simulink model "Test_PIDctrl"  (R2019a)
settings: Solver=VariableStepAuto  StartTime=0.0  StopTime=50  RelTol=1e-3
InitFcn:
  | Test_LibVishia_Ctrl.Test_PIDctrl_init();
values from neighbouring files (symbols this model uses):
  Tstep = 0.000050    (= 5e-05)    [TestOrthOsc_init.m]    (also in Test_PIDctrl_init.m = 0.0001)
libraries: libVishia_CtrlSfn x8, libVishia_Ctrl x3

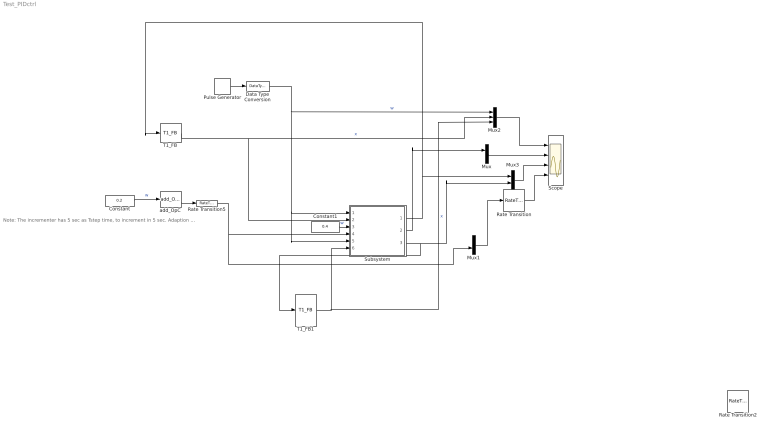
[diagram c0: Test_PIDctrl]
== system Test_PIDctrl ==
  note: Note: The incrementer has 5 sec as Tstep time, to increment in 5 sec. Adaption to Tparam with rate transition.
  Constant : Constant  Value=0.2  OutDataTypeStr=single  SampleTime=5
  Constant1 : Constant  Value=0.4  OutDataTypeStr=single  SampleTime=7.5
  Data Type Conversion : DataTypeConversion  OutDataTypeStr=single
  Mux : Mux  Inputs=2
  Mux1 : Mux  Inputs=2
  Mux2 : Mux  Inputs=3
  Mux3 : Mux  Inputs=2
  Pulse Generator : DiscretePulseGenerator  PulseType=Time based  Amplitude=0.1  Period=5  PulseWidth=50
  Rate Transition : RateTransition  OutPortSampleTime=Tstep
  Rate Transition2 : RateTransition  OutPortSampleTime=Tstep
  Rate Transition5 : RateTransition  OutPortSampleTime=Tparam
  Scope : Scope  NumInputPorts=4
  Subsystem : Subsystem
  T1_FB : libVishia_Ctrl/T1_FB  T1=0.5  y0=0  Tstep=Tstep
  T1_FB1 : libVishia_Ctrl/T1_FB  T1=0.5  y0=0  Tstep=Tstep
  add_OpC : libVishia_Ctrl/add_OpC  y0=0
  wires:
  T1_FB/2 -> Subsystem/2(x), Mux2/2  "x"
  Mux/1 -> Scope/2
  Pulse Generator/1 -> Data Type Conversion/1
  add_OpC/2 -> Rate Transition5/1
  Constant/1 -> add_OpC/1  "w"
  Rate Transition/1 -> Scope/4
  Mux1/1 -> Rate Transition/1
  Subsystem/1(y) -> T1_FB/1, Mux3/1
  Data Type Conversion/1 -> Mux2/1, Subsystem/5(w1), Subsystem/1(w)  "w"
  Subsystem/2(Out1) -> Mux/1
  Constant1/1 -> Subsystem/3(yLim)  "w"
  Mux2/1 -> Scope/1
  Subsystem/3(y1) -> T1_FB1/1, Mux3/2
  Mux3/1 -> Scope/3
  T1_FB1/2 -> Mux2/3, Subsystem/6(x1)  "x"
  Rate Transition5/1 -> Subsystem/4(kP), Mux1/2

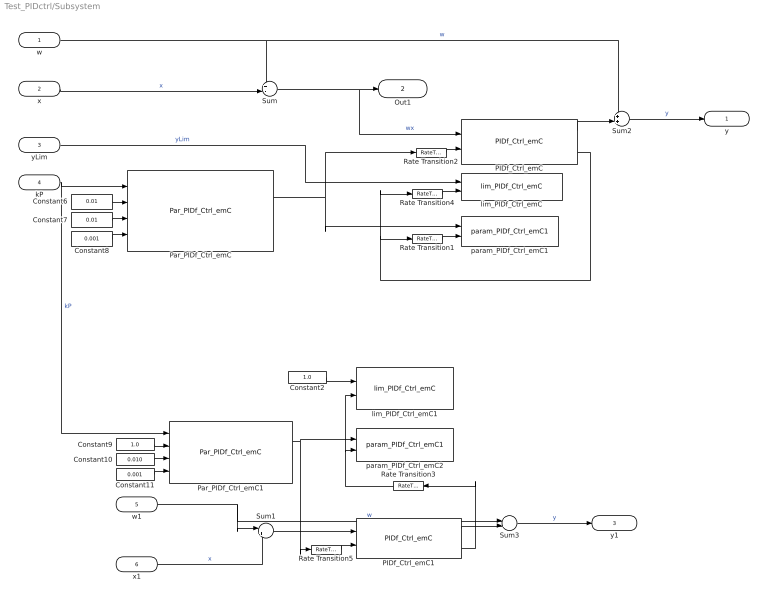
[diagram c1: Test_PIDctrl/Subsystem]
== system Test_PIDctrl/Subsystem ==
  w : Inport  SampleTime=Tstep
  x : Inport  Port=2
  yLim : Inport  Port=3
  kP : Inport  Port=4
  w1 : Inport  Port=5  SampleTime=Tstep
  x1 : Inport  Port=6
  Constant10 : Constant  Value=0.010  OutDataTypeStr=single  SampleTime=-1
  Constant11 : Constant  Value=0.001  OutDataTypeStr=single  SampleTime=-1
  Constant2 : Constant  Value=1.0  OutDataTypeStr=single  SampleTime=-1
  Constant6 : Constant  Value=0.01  OutDataTypeStr=single  SampleTime=-1
  Constant7 : Constant  Value=0.01  OutDataTypeStr=single  SampleTime=-1
  Constant8 : Constant  Value=0.001  OutDataTypeStr=single  SampleTime=-1
  Constant9 : Constant  Value=1.0  OutDataTypeStr=single  SampleTime=-1
  PIDf_Ctrl_emC : libVishia_CtrlSfn/PIDf_Ctrl_emC  Tstep=Tstep
  PIDf_Ctrl_emC1 : libVishia_CtrlSfn/PIDf_Ctrl_emC  Tstep=Tstep
  Par_PIDf_Ctrl_emC : libVishia_CtrlSfn/Par_PIDf_Ctrl_emC  Tparam=Tparam  Tctrl=Tstep  yMax=1.2
  Par_PIDf_Ctrl_emC1 : libVishia_CtrlSfn/Par_PIDf_Ctrl_emC  Tparam=0.1  Tctrl=Tstep  yMax=1.2
  Rate Transition1 : RateTransition  OutPortSampleTimeOpt=Inherit  OutPortSampleTime=1.0
  Rate Transition2 : RateTransition  OutPortSampleTimeOpt=Inherit  OutPortSampleTime=Tinit
  Rate Transition3 : RateTransition  OutPortSampleTimeOpt=Inherit  OutPortSampleTime=1.0
  Rate Transition4 : RateTransition  OutPortSampleTimeOpt=Inherit  OutPortSampleTime=4.0
  Rate Transition5 : RateTransition  OutPortSampleTimeOpt=Inherit  OutPortSampleTime=Tinit
  Sum : Sum  Inputs=+-|
  Sum1 : Sum  Inputs=|+-
  Sum2 : Sum  Inputs=++|
  Sum3 : Sum  Inputs=++|
  lim_PIDf_Ctrl_emC : libVishia_CtrlSfn/lim_PIDf_Ctrl_emC
  lim_PIDf_Ctrl_emC1 : libVishia_CtrlSfn/lim_PIDf_Ctrl_emC
  param_PIDf_Ctrl_emC1 : libVishia_CtrlSfn/param_PIDf_Ctrl_emC1
  param_PIDf_Ctrl_emC2 : libVishia_CtrlSfn/param_PIDf_Ctrl_emC1
  y : Outport
  Out1 : Outport  Port=2
  y1 : Outport  Port=3
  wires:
  Sum/1 -> Out1/1, PIDf_Ctrl_emC/1  "wx"
  Par_PIDf_Ctrl_emC/1 -> Rate Transition2/1, param_PIDf_Ctrl_emC1/1
  yLim/1 -> lim_PIDf_Ctrl_emC/1  "yLim"
  w/1 -> Sum/1, Sum2/1  "w"
  Constant6/1 -> Par_PIDf_Ctrl_emC/2
  PIDf_Ctrl_emC/3 -> Rate Transition4/1, Rate Transition1/1
  Constant8/1 -> Par_PIDf_Ctrl_emC/4
  Rate Transition4/1 -> lim_PIDf_Ctrl_emC/2
  PIDf_Ctrl_emC/1 -> Sum2/2
  Rate Transition1/1 -> param_PIDf_Ctrl_emC1/2
  Constant7/1 -> Par_PIDf_Ctrl_emC/3
  Sum2/1 -> y/1  "y"
  kP/1 -> Par_PIDf_Ctrl_emC1/1, Par_PIDf_Ctrl_emC/1  "kP"
  x/1 -> Sum/2  "x"
  Rate Transition2/1 -> PIDf_Ctrl_emC/2
  w1/1 -> Sum3/1, Sum1/1  "w"
  Par_PIDf_Ctrl_emC1/1 -> Rate Transition5/1, param_PIDf_Ctrl_emC2/1
  Constant2/1 -> lim_PIDf_Ctrl_emC1/1
  x1/1 -> Sum1/2  "x"
  Constant11/1 -> Par_PIDf_Ctrl_emC1/4
  Constant10/1 -> Par_PIDf_Ctrl_emC1/3
  Sum1/1 -> PIDf_Ctrl_emC1/1
  PIDf_Ctrl_emC1/3 -> Rate Transition3/1
  Constant9/1 -> Par_PIDf_Ctrl_emC1/2
  Sum3/1 -> y1/1  "y"
  PIDf_Ctrl_emC1/1 -> Sum3/2
  Rate Transition3/1 -> lim_PIDf_Ctrl_emC1/2, param_PIDf_Ctrl_emC2/2
  Rate Transition5/1 -> PIDf_Ctrl_emC1/2
